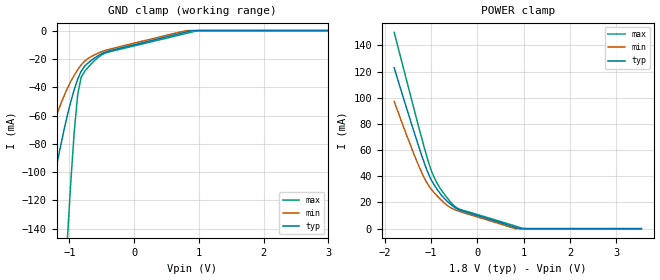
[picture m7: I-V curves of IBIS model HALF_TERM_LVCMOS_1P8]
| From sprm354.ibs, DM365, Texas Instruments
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|   Model Cell HALF_TERM_LVCMOS_1P8
|HALF_TERM_LVCMOS_1P8
[Model]   HALF_TERM_LVCMOS_1P8
Model_type   Input
Polarity   Non-Inverting
Vinl =  0.63
Vinh =  1.17
C_comp   3.009089p   2.23501p   3.950269p
[Model Spec]
Vinl   0.63   0.567   0.693
Vinh   1.17   1.053   1.287
[Temperature Range]   25   125   -40
[Voltage Range]   1.8   1.62   1.98
[POWER_clamp]
|   voltage   I(typ)   I(min)   I(max)
-1.8V     122.9mA    97.15mA    149.9mA
-1.309V   67.07mA    51.4mA     82.96mA
-1.145V   49.82mA    38.47mA    61.37mA
-1.036V   40.01mA    31.91mA    48.32mA
-927.3mV  32.91mA    27.11mA    38.47mA
-818.2mV  27.38mA    23.02mA    31.47mA
-654.5mV  20.99mA    17.75mA    23.46mA
-490.9mV  16.21mA    14.49mA    17.07mA
-327.3mV  13.47mA    12.44mA    14.19mA
818.2mV   986.3uA    9.608uA    1.978mA
981.8mV   0A         0A         178.9uA
3.545V    0A         0A         0A
[GND_clamp]
|   voltage   I(typ)   I(min)   I(max)
-1.8V     -238.9mA   -142.6mA   -823.4mA
-1.418V   -146.7mA   -88.57mA   -482.7mA
-1.364V   -133.7mA   -81.17mA   -433.9mA
-1.036V   -60.59mA   -41.19mA   -150.4mA
-981.8mV  -50.58mA   -36.09mA   -108.6mA
-927.3mV  -41.77mA   -31.59mA   -71.93mA
-872.7mV  -34.29mA   -27.63mA   -44.96mA
-818.2mV  -28.61mA   -24.22mA   -32.85mA
-654.5mV  -20.75mA   -18.09mA   -23.11mA
-436.4mV  -15.06mA   -13.89mA   -15.76mA
981.8mV   0A         0A         -1.329uA
3.545V    0A         0A         0A
